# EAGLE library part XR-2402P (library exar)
V.22bis high perfomance AFE
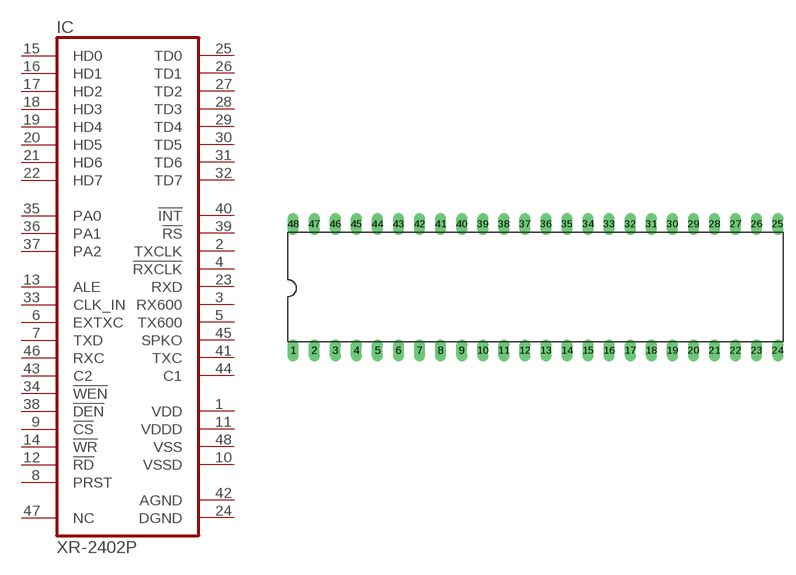
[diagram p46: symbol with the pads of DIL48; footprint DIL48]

Designator prefix IC

## XR-2402P (OC_FARNELL: unknown; OC_NEWARK: unknown)  [DIL48]
1  VDD  pwr
2  TXCLK  out
3  RX600  out
4  !RXCLK  out
5  TX600  out
6  EXTXC  in
7  TXD  in
8  PRST  in
9  !CS  in
10  VSSD  pwr
11  VDDD  pwr
12  !RD  in
13  ALE  in
14  !WR  in
15  HD0
16  HD1
17  HD2
18  HD3
19  HD4
20  HD5
21  HD6
22  HD7
23  RXD  out
24  DGND  pwr
25  TD0
26  TD1
27  TD2
28  TD3
29  TD4
30  TD5
31  TD6
32  TD7
33  CLK_IN  in
34  !WEN  in
35  PA0  in
36  PA1  in
37  PA2  in
38  !DEN  in
39  !RS  out
40  !INT  out
41  TXC  out
42  AGND  pwr
43  C2  in
44  C1  out
45  SPKO  out
46  RXC  in
47  NC  nc
48  VSS  pwr

## Footprint DIL48 (pad centres in mm)
Dual In Line Package
drill 0.813 long: 1 -29.21,-7.62; 2 -26.67,-7.62; 3 -24.13,-7.62; 4 -21.59,-7.62; 5 -19.05,-7.62; 6 -16.51,-7.62; 7 -13.97,-7.62; 8 -11.43,-7.62; 9 -8.89,-7.62; 10 -6.35,-7.62; 11 -3.81,-7.62; 12 -1.27,-7.62; 13 1.27,-7.62; 14 3.81,-7.62; 15 6.35,-7.62; 16 8.89,-7.62; 17 11.43,-7.62; 18 13.97,-7.62; 19 16.51,-7.62; 20 19.05,-7.62; 21 21.59,-7.62; 22 24.13,-7.62; 23 26.67,-7.62; 24 29.21,-7.62; 25 29.21,7.62; 26 26.67,7.62; 27 24.13,7.62; 28 21.59,7.62; 29 19.05,7.62; 30 16.51,7.62; 31 13.97,7.62; 32 11.43,7.62; 33 8.89,7.62; 34 6.35,7.62; 35 3.81,7.62; 36 1.27,7.62; 37 -1.27,7.62; 38 -3.81,7.62; 39 -6.35,7.62; 40 -8.89,7.62; 41 -11.43,7.62; 42 -13.97,7.62; 43 -16.51,7.62; 44 -19.05,7.62; 45 -21.59,7.62; 46 -24.13,7.62; 47 -26.67,7.62; 48 -29.21,7.62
